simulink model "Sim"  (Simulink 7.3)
settings: Solver=ode45  StartTime=0.0  StopTime=200  RelTol=1e-3
undefined symbols (not defined in the file or in its folder): Av, Bv, Cv, Dv, Kmix, Kpr, Kq

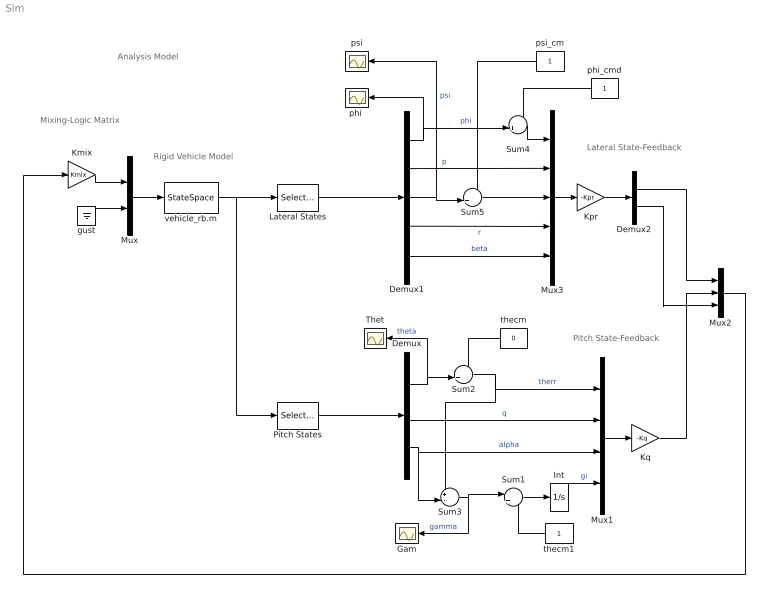
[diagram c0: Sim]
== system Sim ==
  note: Analysis Model
  note: Rigid Vehicle Model
  note: Pitch State-Feedback
  note: Lateral State-Feedback
  note: Mixing-Logic Matrix
  Demux : Demux  Outputs=3
  Demux1 : Demux  Outputs=5
  Demux2 : Demux  Outputs=2
  Gam : Scope
  Int : Integrator
  Kmix : Gain  Gain=Kmix  Multiplication=Matrix(K*u)  ParameterDataType=fixdt(1, 16)  ParameterScaling=2^0  OutDataType=fixdt(1, 16)  OutScaling=2^0
  Kpr : Gain  Gain=-Kpr  Multiplication=Matrix(K*u)  ParameterDataType=fixdt(1, 16)  ParameterScaling=2^0  OutDataType=fixdt(1, 16)  OutScaling=2^0
  Kq : Gain  Gain=-Kq  Multiplication=Matrix(K*u)  ParameterDataType=fixdt(1, 16)  ParameterScaling=2^0  OutDataType=fixdt(1, 16)  OutScaling=2^0
  Lateral States : Selector  InputPortWidth=14  IndexOptions=Index vector (dialog)  Indices=[1,2, 5,6, 8]  OutputSizes=1
  Mux : Mux  Inputs=[4,1]
  Mux1 : Mux
  Mux2 : Mux  Inputs=3
  Mux3 : Mux  Inputs=5
  Pitch States : Selector  InputPortWidth=14  IndexOptions=Index vector (dialog)  Indices=[3, 4, 7]  OutputSizes=1
  Sum1 : Sum  Inputs=|+-  OutDataType=sfix(16)  OutScaling=2^0
  Sum2 : Sum  Inputs=-+|  OutDataType=sfix(16)  OutScaling=2^0
  Sum3 : Sum  Inputs=+-|  OutDataType=sfix(16)  OutScaling=2^0
  Sum4 : Sum  Inputs=-+|  OutDataType=sfix(16)  OutScaling=2^0
  Sum5 : Sum  Inputs=-+|  OutDataType=sfix(16)  OutScaling=2^0
  Thet : Scope
  gust : Ground
  "phi " : Scope
  phi_cmd : Constant  OutDataType=fixdt(1, 16)  OutScaling=2^0
  psi : Scope
  psi_cm : Constant  OutDataType=fixdt(1, 16)  OutScaling=2^0
  thecm : Constant  Value=0  OutDataType=fixdt(1, 16)  OutScaling=2^0
  thecm1 : Constant  OutDataType=fixdt(1, 16)  OutScaling=2^0
  vehicle_rb.m : StateSpace  A=Av  B=Bv  C=Cv  D=Dv
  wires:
  Mux/1 -> vehicle_rb.m/1
  Kmix/1 -> Mux/1
  gust/1 -> Mux/2
  vehicle_rb.m/1 -> Pitch States/1, Lateral States/1
  Demux/2 -> Mux1/2  "q"
  Demux/3 -> Mux1/3, Sum3/2  "alpha"
  Pitch States/1 -> Demux/1
  Mux1/1 -> Kq/1
  Demux/1 -> Sum2/2, Thet/1  "theta"
  Sum2/1 -> Mux1/1, Sum3/1  "therr"
  thecm/1 -> Sum2/1
  Kq/1 -> Mux2/2
  Int/1 -> Mux1/4  "gi"
  thecm1/1 -> Sum1/2
  Sum1/1 -> Int/1
  Sum3/1 -> Sum1/1, Gam/1  "gamma"
  Demux1/2 -> Mux3/2  "p"
  Lateral States/1 -> Demux1/1
  Mux3/1 -> Kpr/1
  Demux1/4 -> Mux3/4  "r"
  psi_cm/1 -> Sum5/1
  Demux1/5 -> Mux3/5  "beta"
  Demux1/3 -> Sum5/2, psi/1  "psi"
  Sum5/1 -> Mux3/3
  Kpr/1 -> Demux2/1
  Demux2/1 -> Mux2/1
  Demux2/2 -> Mux2/3
  Sum4/1 -> Mux3/1
  Demux1/1 -> Sum4/2, "phi "/1  "phi"
  phi_cmd/1 -> Sum4/1
  Mux2/1 -> Kmix/1
